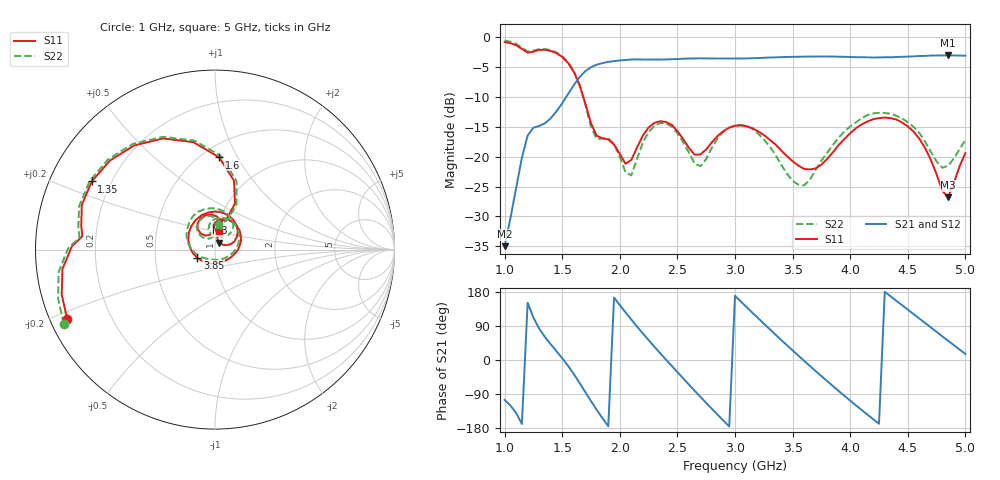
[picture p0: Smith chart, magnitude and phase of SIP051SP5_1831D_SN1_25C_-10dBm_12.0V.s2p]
# GHz  S  dB  R  50
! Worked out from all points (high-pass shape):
!   81 points, 1 GHz to 5 GHz, reference 50 ohm
!   highest |S21| = -3.04 dB at 4.85 GHz (marker M1); lowest = -35.0 dB at 1 GHz (marker M2)
!   |S21| within 3 dB of the highest: 1.683 GHz to end of sweep
!   lowest |S11| = -26.8 dB at 4.85 GHz (marker M3), VSWR 1.10, Z = 52.3 + j4.05 ohm
!   |S11| at or under -10 dB: 1.683 GHz to end of sweep
!   |S22| runs from -24.8 to -0.5 dB; largest |S21 - S12| = 0.0027
!   S11 on the Smith chart (normalised r, x): 1 GHz: 0.05, -0.22; 1.35 GHz: 0.13, +0.25; 1.6 GHz: 0.60, +0.84; 3.85 GHz: 0.82, -0.07; 5 GHz: 1.02, +0.22
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1  -0.82 -154.8  -34.98 -105.3  -35.13 -104.7  -0.55 -153.9
1.2  -2.58 174.3  -16.45 151.2  -16.48 151.4  -2.41 175.0
1.35  -2.10 151.1  -14.41 60.8  -14.42 60.8  -1.99 151.4
1.6  -5.78 87.4  -8.03 -36.8  -8.04 -36.8  -5.67 86.0
1.7  -11.04 66.6  -5.70 -84.3  -5.70 -84.3  -11.20 64.3
1.85  -16.91 90.1  -4.33 -153.8  -4.32 -153.8  -16.95 91.8
1.95  -17.97 90.6  -4.00 164.7  -4.00 164.8  -17.87 87.4
2.15  -18.45 131.6  -3.72 88.2  -3.72 88.2  -20.32 135.6
2.35  -14.07 104.9  -3.74 18.1  -3.73 18.2  -14.38 109.6
2.5  -15.71 79.0  -3.66 -31.8  -3.65 -31.8  -16.09 79.7
2.65  -19.67 80.2  -3.56 -81.2  -3.55 -81.1  -21.18 78.6
2.85  -16.51 90.2  -3.57 -144.8  -3.56 -144.7  -16.90 103.1
3  -14.81 66.8  -3.57 169.5  -3.56 169.6  -14.80 76.1
3.3  -17.15 8.8  -3.40 81.7  -3.40 81.7  -18.26 4.8
3.5  -20.76 -33.7  -3.29 25.4  -3.29 25.4  -24.05 -61.4
3.7  -21.95 -100.0  -3.23 -29.2  -3.23 -29.1  -22.21 -142.7
3.85  -19.27 -155.4  -3.24 -68.8  -3.24 -68.8  -18.03 -178.0
4.05  -15.24 147.6  -3.35 -119.6  -3.33 -119.6  -14.25 142.5
4.35  -13.55 78.2  -3.36 168.1  -3.36 168.2  -12.81 87.2
4.6  -17.00 30.3  -3.15 109.5  -3.16 109.5  -16.02 50.3
4.85  -26.80 57.6  -3.04 50.7  -3.05 50.8  -21.53 74.7
5  -19.40 78.5  -3.10 16.0  -3.11 16.1  -17.22 81.0
